(* Logix 5000 AddOnInstructionDefinition export Banner_LE_Param_v4; software revision 33.00; part 2 of 2 *)
(* tags used below, declared in another part *)
   LE : Banner_LE_v4;
   Port_Data : Banner_IOL_Port_v4;
   Port : DINT;
   Local_Control : DINT;
   Command_Being_Processed : BOOL;
   Update_Archive : BOOL;
   Index_Write_Control : DINT;
   Index_Write_Inprocess : INT;
   Inprocess_Index : DINT;
(* Banner_LE_Param_v4, continued *)

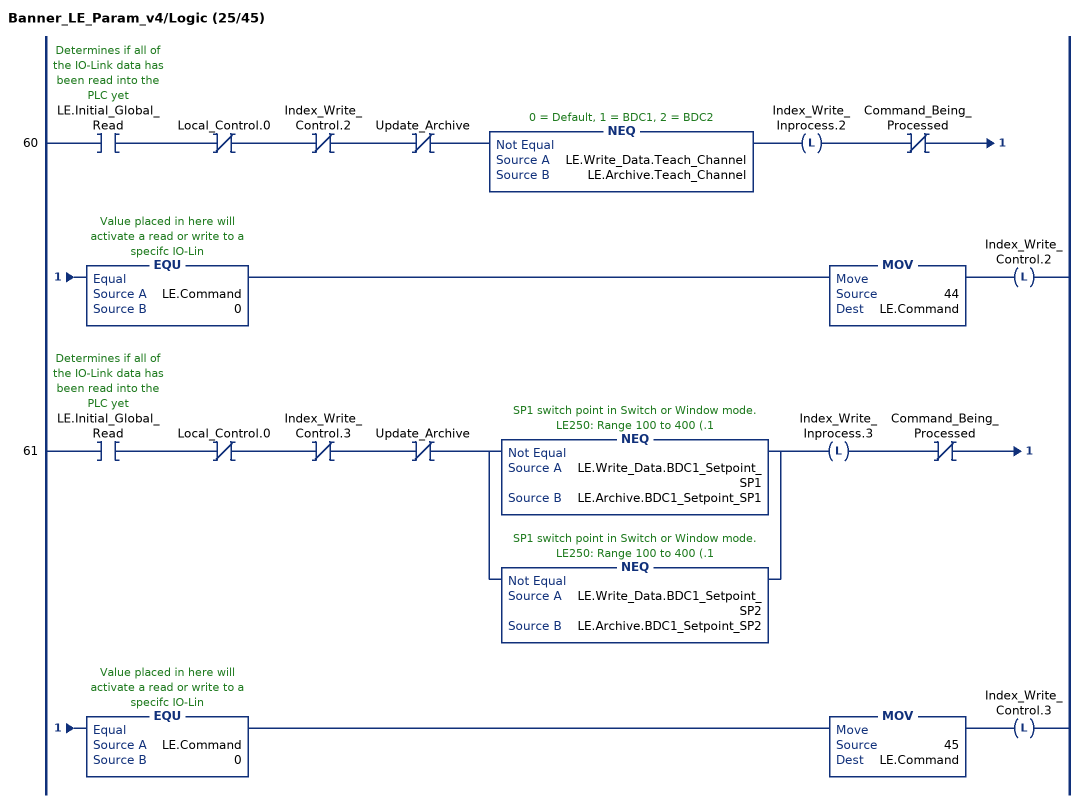
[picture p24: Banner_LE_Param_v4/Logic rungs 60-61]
   60: XIC(LE.Initial_Global_Read)XIO(Local_Control.0)XIO(Index_Write_Control.2)XIO(Update_Archive)NEQ(LE.Write_Data.Teach_Channel,LE.Archive.Teach_Channel)OTL(Index_Write_Inprocess.2)XIO(Command_Being_Processed)EQU(LE.Command,0)MOV(44,LE.Command)OTL(Index_Write_Control.2);
   61: XIC(LE.Initial_Global_Read)XIO(Local_Control.0)XIO(Index_Write_Control.3)XIO(Update_Archive)[NEQ(LE.Write_Data.BDC1_Setpoint_SP1,LE.Archive.BDC1_Setpoint_SP1) ,NEQ(LE.Write_Data.BDC1_Setpoint_SP2,LE.Archive.BDC1_Setpoint_SP2) ]OTL(Index_Write_Inprocess.3)XIO(Command_Being_Processed)EQU(LE.Command,0)MOV(45,LE.Command)OTL(Index_Write_Control.3);
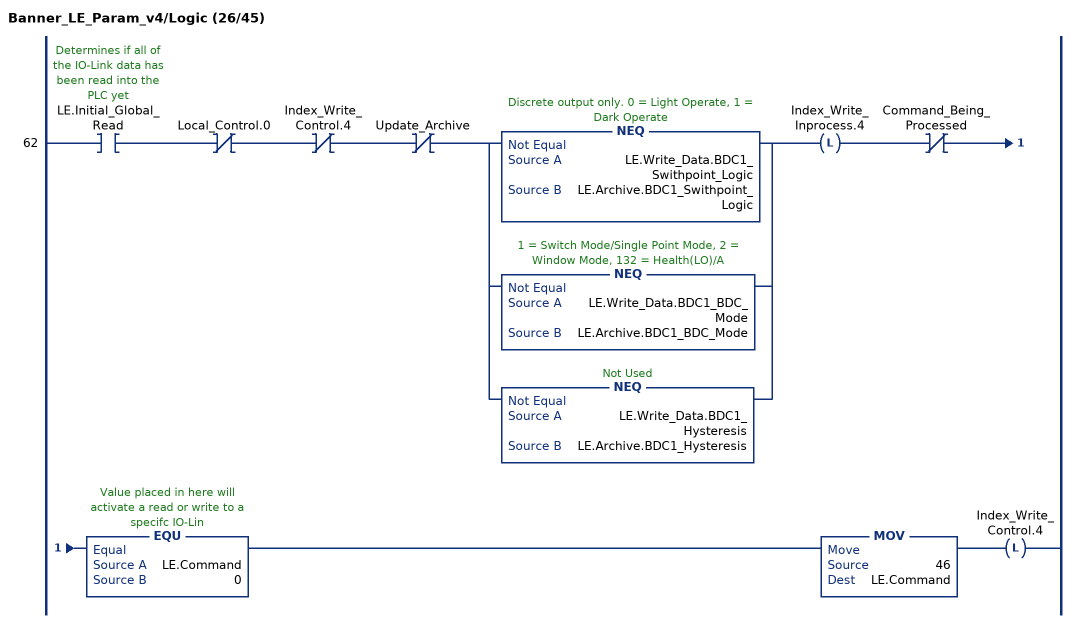
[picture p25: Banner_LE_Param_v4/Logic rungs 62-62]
   62: XIC(LE.Initial_Global_Read)XIO(Local_Control.0)XIO(Index_Write_Control.4)XIO(Update_Archive)[NEQ(LE.Write_Data.BDC1_Swithpoint_Logic,LE.Archive.BDC1_Swithpoint_Logic) ,NEQ(LE.Write_Data.BDC1_BDC_Mode,LE.Archive.BDC1_BDC_Mode) ,NEQ(LE.Write_Data.BDC1_Hysteresis,LE.Archive.BDC1_Hysteresis) ]OTL(Index_Write_Inprocess.4)XIO(Command_Being_Processed)EQU(LE.Command,0)MOV(46,LE.Command)OTL(Index_Write_Control.4);
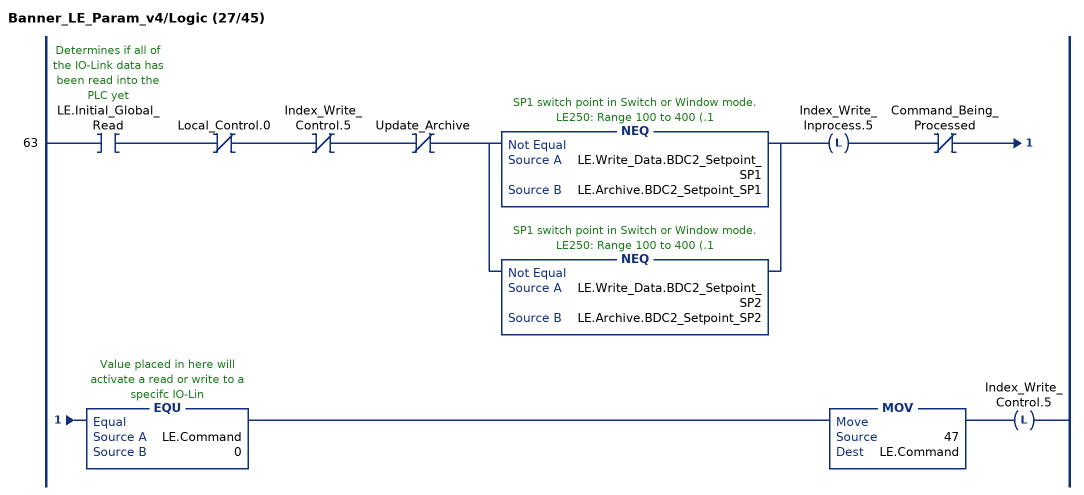
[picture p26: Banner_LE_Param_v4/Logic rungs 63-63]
   63: XIC(LE.Initial_Global_Read)XIO(Local_Control.0)XIO(Index_Write_Control.5)XIO(Update_Archive)[NEQ(LE.Write_Data.BDC2_Setpoint_SP1,LE.Archive.BDC2_Setpoint_SP1) ,NEQ(LE.Write_Data.BDC2_Setpoint_SP2,LE.Archive.BDC2_Setpoint_SP2) ]OTL(Index_Write_Inprocess.5)XIO(Command_Being_Processed)EQU(LE.Command,0)MOV(47,LE.Command)OTL(Index_Write_Control.5);
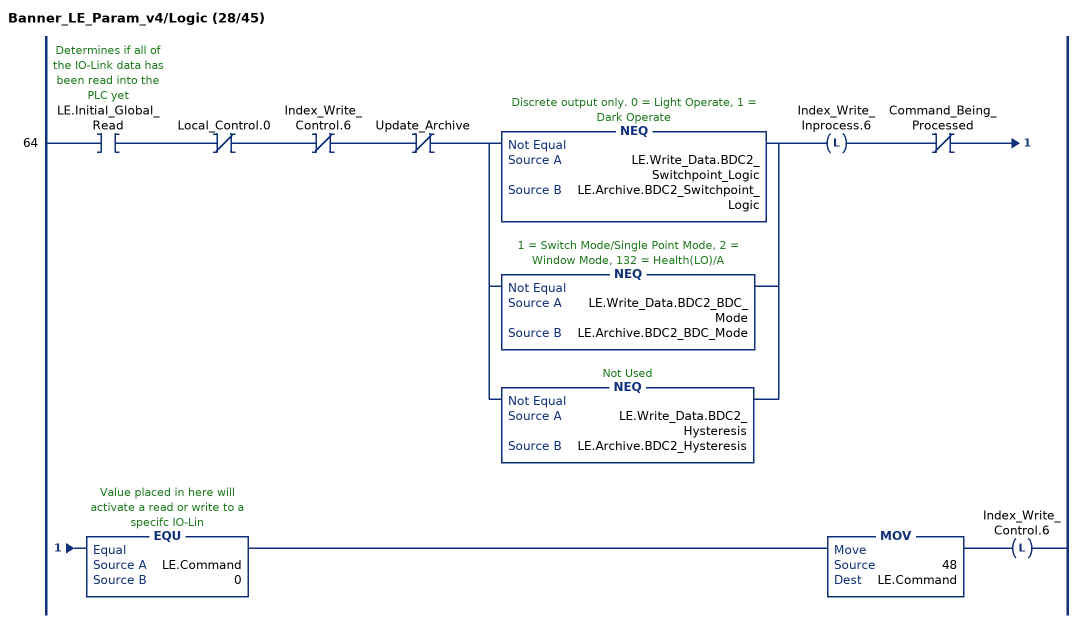
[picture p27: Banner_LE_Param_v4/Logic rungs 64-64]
   64: XIC(LE.Initial_Global_Read)XIO(Local_Control.0)XIO(Index_Write_Control.6)XIO(Update_Archive)[NEQ(LE.Write_Data.BDC2_Switchpoint_Logic,LE.Archive.BDC2_Switchpoint_Logic) ,NEQ(LE.Write_Data.BDC2_BDC_Mode,LE.Archive.BDC2_BDC_Mode) ,NEQ(LE.Write_Data.BDC2_Hysteresis,LE.Archive.BDC2_Hysteresis) ]OTL(Index_Write_Inprocess.6)XIO(Command_Being_Processed)EQU(LE.Command,0)MOV(48,LE.Command)OTL(Index_Write_Control.6);
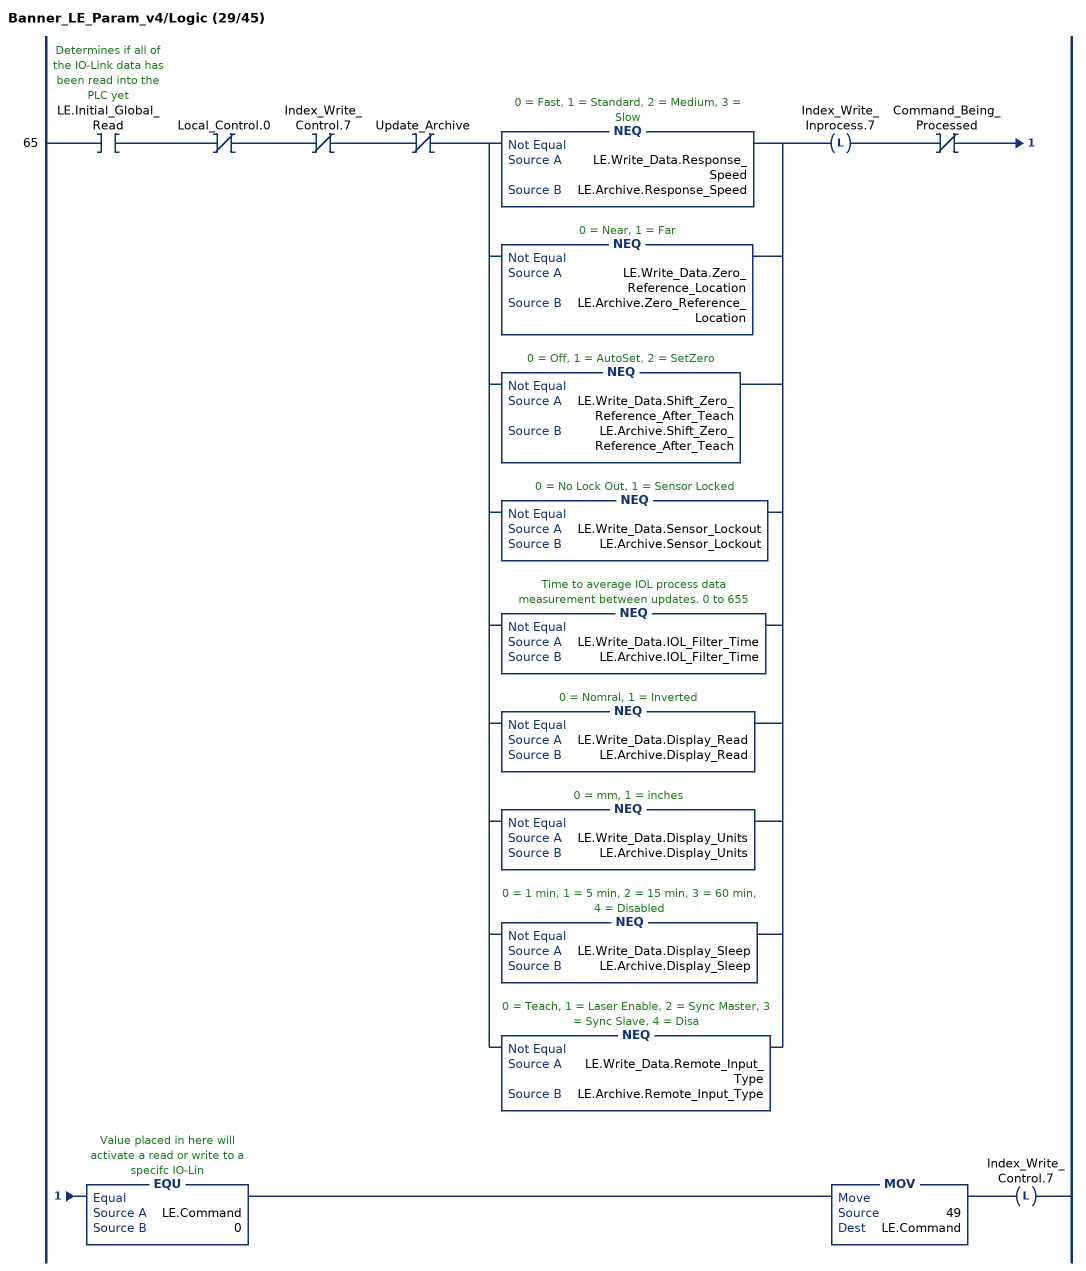
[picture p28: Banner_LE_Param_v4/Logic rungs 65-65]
   65: XIC(LE.Initial_Global_Read)XIO(Local_Control.0)XIO(Index_Write_Control.7)XIO(Update_Archive)[NEQ(LE.Write_Data.Response_Speed,LE.Archive.Response_Speed) ,NEQ(LE.Write_Data.Zero_Reference_Location,LE.Archive.Zero_Reference_Location) ,NEQ(LE.Write_Data.Shift_Zero_Reference_After_Teach,LE.Archive.Shift_Zero_Reference_After_Teach) ,NEQ(LE.Write_Data.Sensor_Lockout,LE.Archive.Sensor_Lockout) ,NEQ(LE.Write_Data.IOL_Filter_Time,LE.Archive.IOL_Filter_Time) ,NEQ(LE.Write_Data.Display_Read,LE.Archive.Display_Read) ,NEQ(LE.Write_Data.Display_Units,LE.Archive.Display_Units) ,NEQ(LE.Write_Data.Display_Sleep,LE.Archive.Display_Sleep) ,NEQ(LE.Write_Data.Remote_Input_Type,LE.Archive.Remote_Input_Type) ]OTL(Index_Write_Inprocess.7)XIO(Command_Being_Processed)EQU(LE.Command,0)MOV(49,LE.Command)OTL(Index_Write_Control.7);
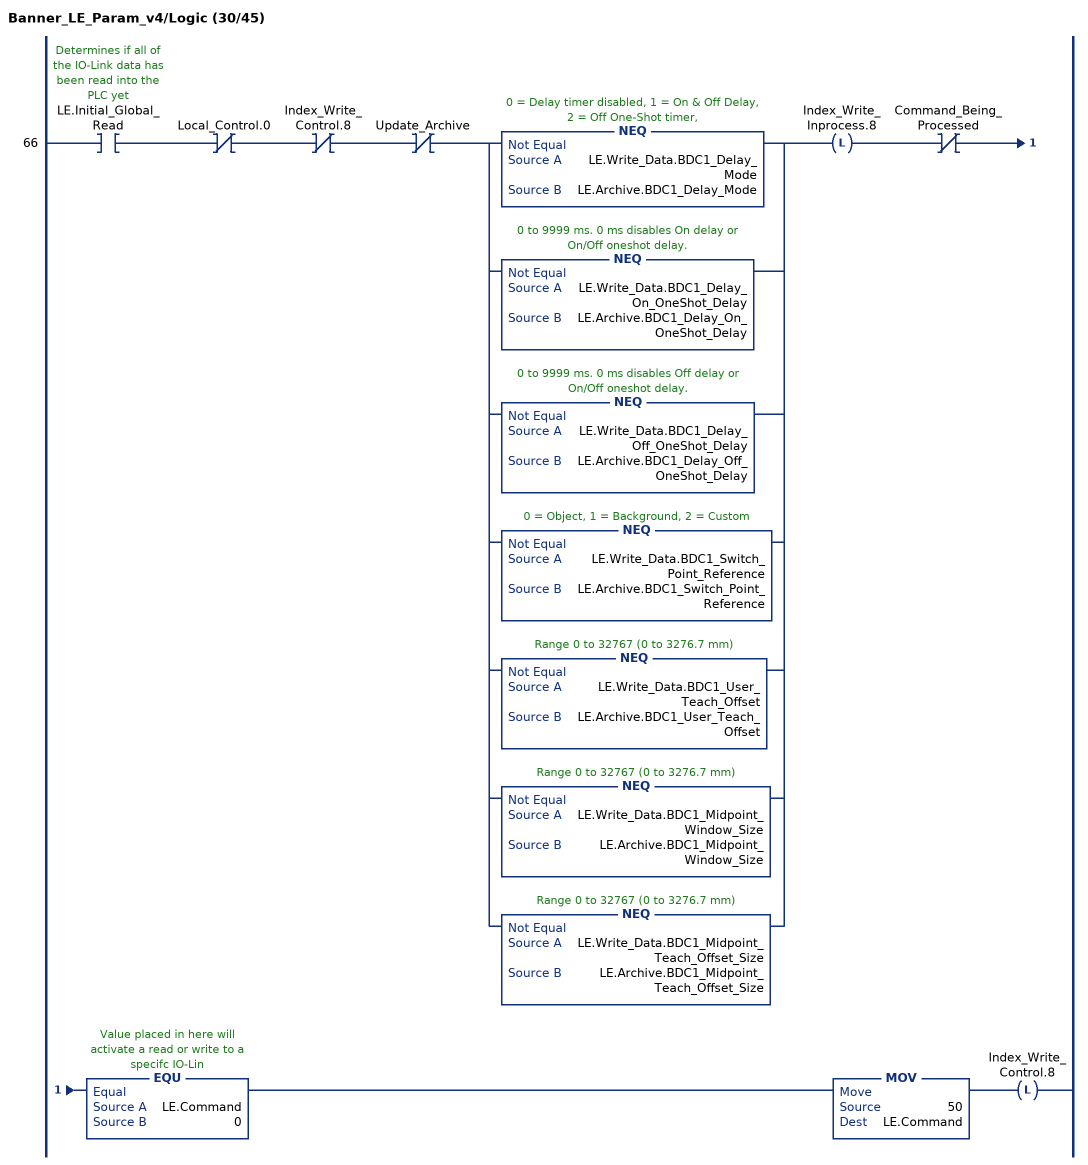
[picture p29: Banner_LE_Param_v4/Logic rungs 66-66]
   66: XIC(LE.Initial_Global_Read)XIO(Local_Control.0)XIO(Index_Write_Control.8)XIO(Update_Archive)[NEQ(LE.Write_Data.BDC1_Delay_Mode,LE.Archive.BDC1_Delay_Mode) ,NEQ(LE.Write_Data.BDC1_Delay_On_OneShot_Delay,LE.Archive.BDC1_Delay_On_OneShot_Delay) ,NEQ(LE.Write_Data.BDC1_Delay_Off_OneShot_Delay,LE.Archive.BDC1_Delay_Off_OneShot_Delay) ,NEQ(LE.Write_Data.BDC1_Switch_Point_Reference,LE.Archive.BDC1_Switch_Point_Reference) ,NEQ(LE.Write_Data.BDC1_User_Teach_Offset,LE.Archive.BDC1_User_Teach_Offset) ,NEQ(LE.Write_Data.BDC1_Midpoint_Window_Size,LE.Archive.BDC1_Midpoint_Window_Size) ,NEQ(LE.Write_Data.BDC1_Midpoint_Teach_Offset_Size,LE.Archive.BDC1_Midpoint_Teach_Offset_Size) ]OTL(Index_Write_Inprocess.8)XIO(Command_Being_Processed)EQU(LE.Command,0)MOV(50,LE.Command)OTL(Index_Write_Control.8);
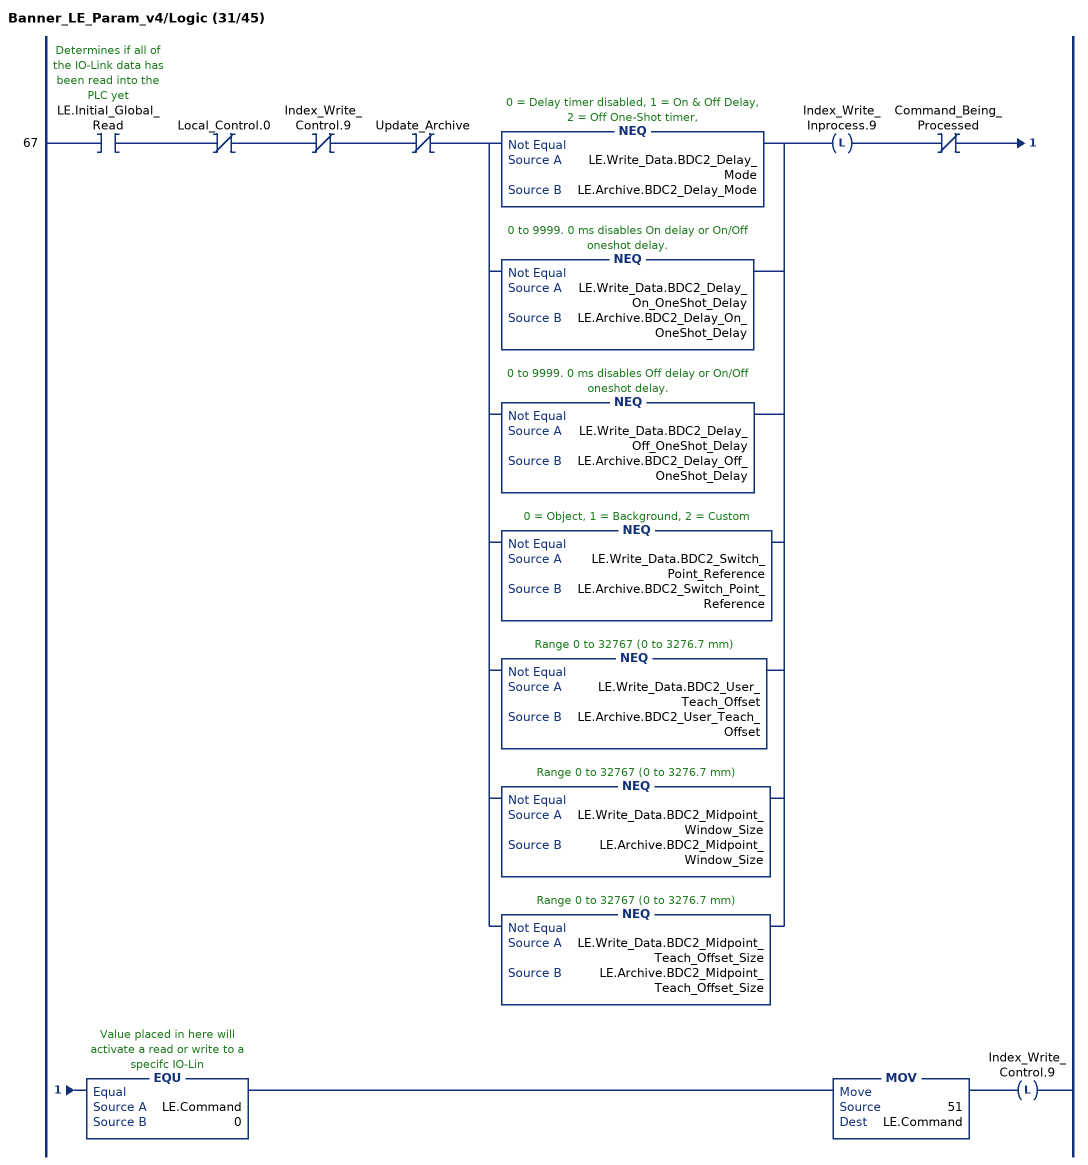
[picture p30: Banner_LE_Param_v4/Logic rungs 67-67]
   67: XIC(LE.Initial_Global_Read)XIO(Local_Control.0)XIO(Index_Write_Control.9)XIO(Update_Archive)[NEQ(LE.Write_Data.BDC2_Delay_Mode,LE.Archive.BDC2_Delay_Mode) ,NEQ(LE.Write_Data.BDC2_Delay_On_OneShot_Delay,LE.Archive.BDC2_Delay_On_OneShot_Delay) ,NEQ(LE.Write_Data.BDC2_Delay_Off_OneShot_Delay,LE.Archive.BDC2_Delay_Off_OneShot_Delay) ,NEQ(LE.Write_Data.BDC2_Switch_Point_Reference,LE.Archive.BDC2_Switch_Point_Reference) ,NEQ(LE.Write_Data.BDC2_User_Teach_Offset,LE.Archive.BDC2_User_Teach_Offset) ,NEQ(LE.Write_Data.BDC2_Midpoint_Window_Size,LE.Archive.BDC2_Midpoint_Window_Size) ,NEQ(LE.Write_Data.BDC2_Midpoint_Teach_Offset_Size,LE.Archive.BDC2_Midpoint_Teach_Offset_Size) ]OTL(Index_Write_Inprocess.9)XIO(Command_Being_Processed)EQU(LE.Command,0)MOV(51,LE.Command)OTL(Index_Write_Control.9);
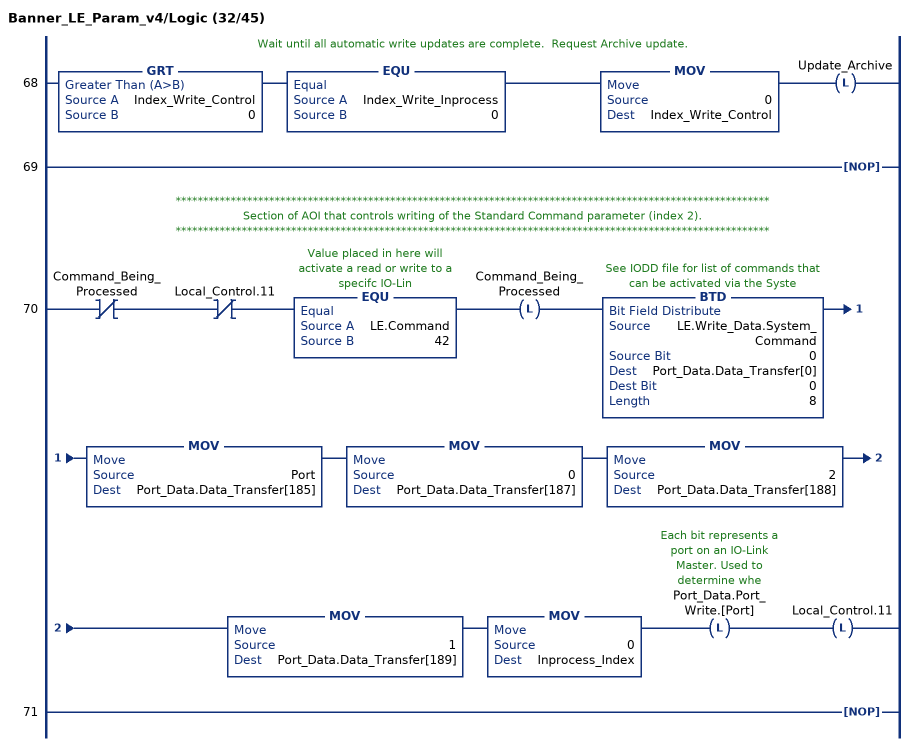
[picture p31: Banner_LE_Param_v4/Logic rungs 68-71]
   // Wait until all automatic write updates are complete.  Request Archive update.
   68: GRT(Index_Write_Control,0)EQU(Index_Write_Inprocess,0)MOV(0,Index_Write_Control)OTL(Update_Archive);
   69: NOP();
   // ************************************************************************************************************
   // Section of AOI that controls writing of the Standard Command parameter (index 2).
   // ************************************************************************************************************
   70: XIO(Command_Being_Processed)XIO(Local_Control.11)EQU(LE.Command,42)OTL(Command_Being_Processed)BTD(LE.Write_Data.System_Command,0,Port_Data.Data_Transfer[0],0,8)MOV(Port,Port_Data.Data_Transfer[185])MOV(0,Port_Data.Data_Transfer[187])MOV(2,Port_Data.Data_Transfer[188])MOV(1,Port_Data.Data_Transfer[189])MOV(0,Inprocess_Index)OTL(Port_Data.Port_Write.[Port])OTL(Local_Control.11);
   71: NOP();
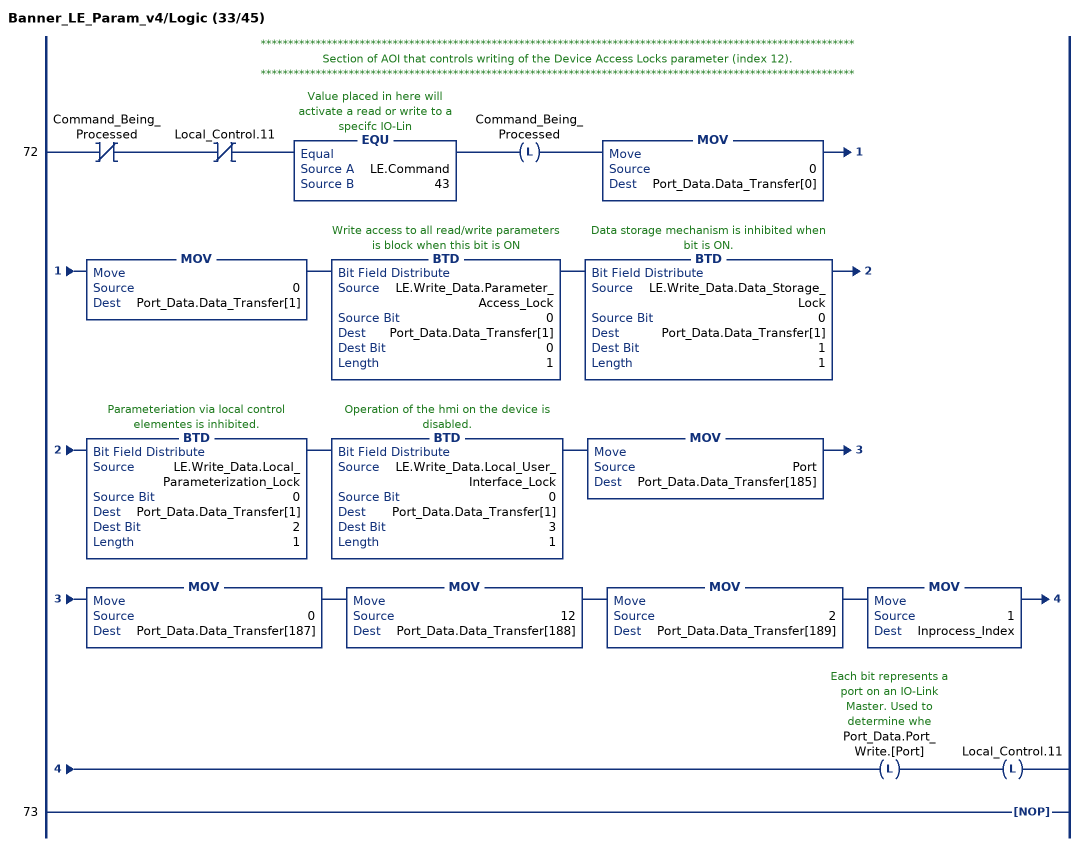
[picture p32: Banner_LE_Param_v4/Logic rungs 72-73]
   // ************************************************************************************************************
   // Section of AOI that controls writing of the Device Access Locks parameter (index 12).
   // ************************************************************************************************************
   72: XIO(Command_Being_Processed)XIO(Local_Control.11)EQU(LE.Command,43)OTL(Command_Being_Processed)MOV(0,Port_Data.Data_Transfer[0])MOV(0,Port_Data.Data_Transfer[1])BTD(LE.Write_Data.Parameter_Access_Lock,0,Port_Data.Data_Transfer[1],0,1)BTD(LE.Write_Data.Data_Storage_Lock,0,Port_Data.Data_Transfer[1],1,1)BTD(LE.Write_Data.Local_Parameterization_Lock,0,Port_Data.Data_Transfer[1],2,1)BTD(LE.Write_Data.Local_User_Interface_Lock,0,Port_Data.Data_Transfer[1],3,1)MOV(Port,Port_Data.Data_Transfer[185])MOV(0,Port_Data.Data_Transfer[187])MOV(12,Port_Data.Data_Transfer[188])MOV(2,Port_Data.Data_Transfer[189])MOV(1,Inprocess_Index)OTL(Port_Data.Port_Write.[Port])OTL(Local_Control.11);
   73: NOP();
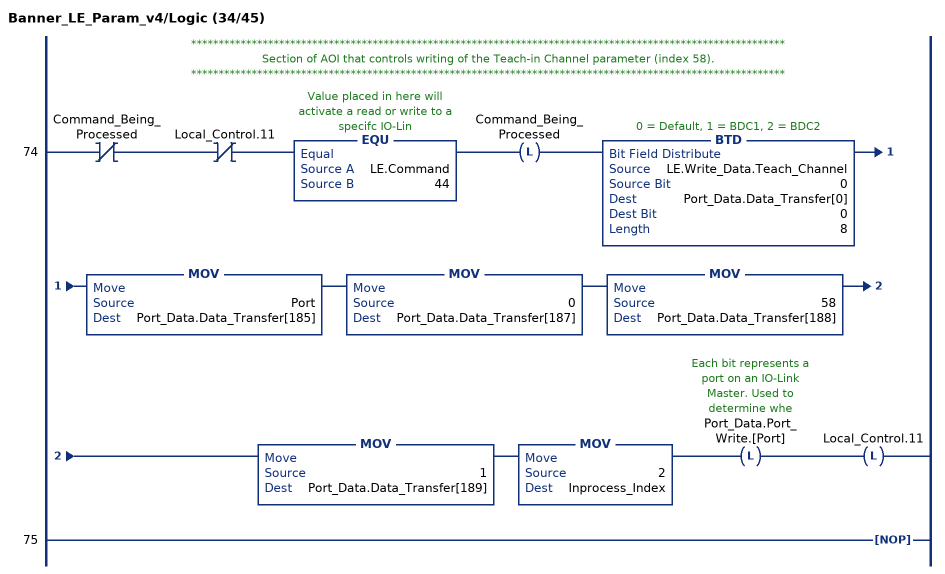
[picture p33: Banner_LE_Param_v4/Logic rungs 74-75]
   // ************************************************************************************************************
   // Section of AOI that controls writing of the Teach-in Channel parameter (index 58).
   // ************************************************************************************************************
   74: XIO(Command_Being_Processed)XIO(Local_Control.11)EQU(LE.Command,44)OTL(Command_Being_Processed)BTD(LE.Write_Data.Teach_Channel,0,Port_Data.Data_Transfer[0],0,8)MOV(Port,Port_Data.Data_Transfer[185])MOV(0,Port_Data.Data_Transfer[187])MOV(58,Port_Data.Data_Transfer[188])MOV(1,Port_Data.Data_Transfer[189])MOV(2,Inprocess_Index)OTL(Port_Data.Port_Write.[Port])OTL(Local_Control.11);
   75: NOP();
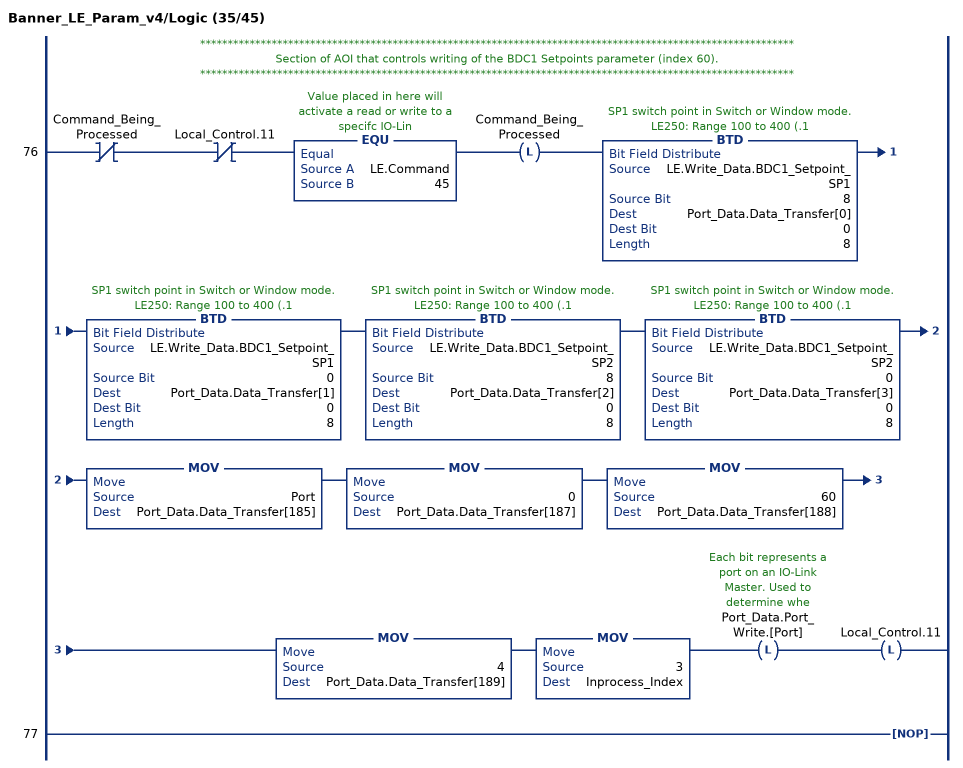
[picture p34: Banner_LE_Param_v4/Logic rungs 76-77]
   // ************************************************************************************************************
   // Section of AOI that controls writing of the BDC1 Setpoints parameter (index 60).
   // ************************************************************************************************************
   76: XIO(Command_Being_Processed)XIO(Local_Control.11)EQU(LE.Command,45)OTL(Command_Being_Processed)BTD(LE.Write_Data.BDC1_Setpoint_SP1,8,Port_Data.Data_Transfer[0],0,8)BTD(LE.Write_Data.BDC1_Setpoint_SP1,0,Port_Data.Data_Transfer[1],0,8)BTD(LE.Write_Data.BDC1_Setpoint_SP2,8,Port_Data.Data_Transfer[2],0,8)BTD(LE.Write_Data.BDC1_Setpoint_SP2,0,Port_Data.Data_Transfer[3],0,8)MOV(Port,Port_Data.Data_Transfer[185])MOV(0,Port_Data.Data_Transfer[187])MOV(60,Port_Data.Data_Transfer[188])MOV(4,Port_Data.Data_Transfer[189])MOV(3,Inprocess_Index)OTL(Port_Data.Port_Write.[Port])OTL(Local_Control.11);
   77: NOP();
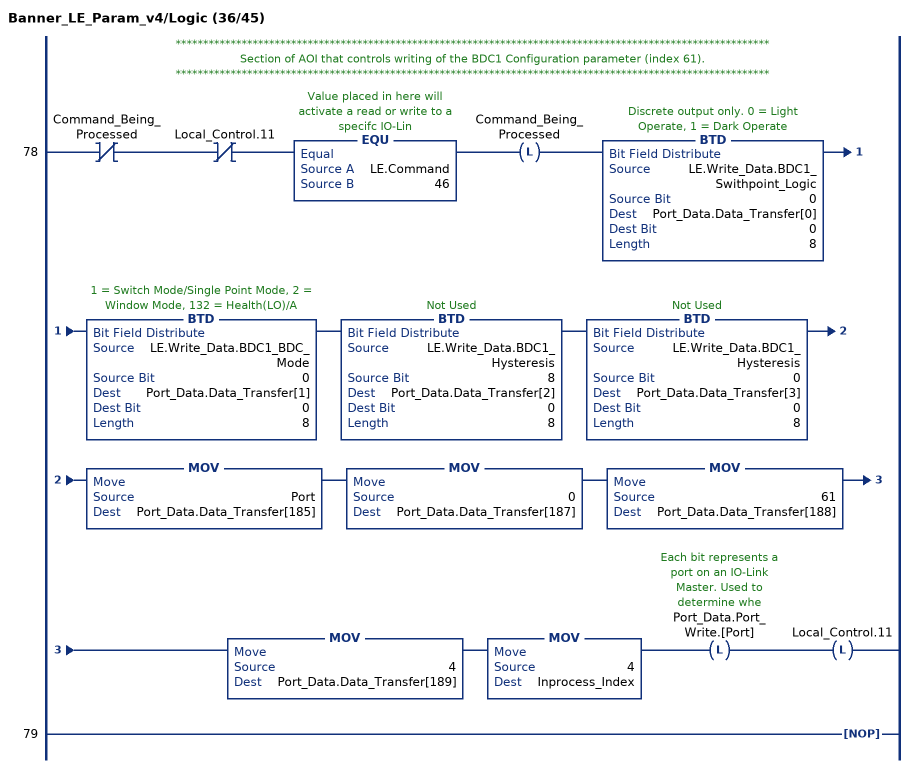
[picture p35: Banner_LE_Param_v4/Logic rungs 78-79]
   // ************************************************************************************************************
   // Section of AOI that controls writing of the BDC1 Configuration parameter (index 61).
   // ************************************************************************************************************
   78: XIO(Command_Being_Processed)XIO(Local_Control.11)EQU(LE.Command,46)OTL(Command_Being_Processed)BTD(LE.Write_Data.BDC1_Swithpoint_Logic,0,Port_Data.Data_Transfer[0],0,8)BTD(LE.Write_Data.BDC1_BDC_Mode,0,Port_Data.Data_Transfer[1],0,8)BTD(LE.Write_Data.BDC1_Hysteresis,8,Port_Data.Data_Transfer[2],0,8)BTD(LE.Write_Data.BDC1_Hysteresis,0,Port_Data.Data_Transfer[3],0,8)MOV(Port,Port_Data.Data_Transfer[185])MOV(0,Port_Data.Data_Transfer[187])MOV(61,Port_Data.Data_Transfer[188])MOV(4,Port_Data.Data_Transfer[189])MOV(4,Inprocess_Index)OTL(Port_Data.Port_Write.[Port])OTL(Local_Control.11);
   79: NOP();
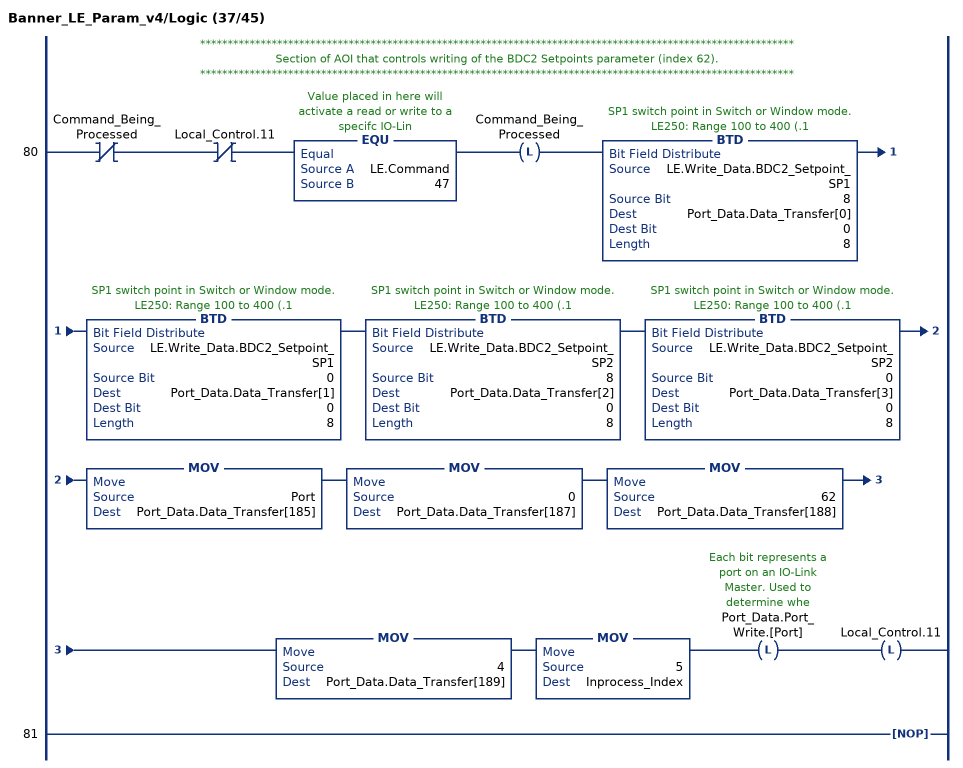
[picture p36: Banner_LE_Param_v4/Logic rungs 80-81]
   // ************************************************************************************************************
   // Section of AOI that controls writing of the BDC2 Setpoints parameter (index 62).
   // ************************************************************************************************************
   80: XIO(Command_Being_Processed)XIO(Local_Control.11)EQU(LE.Command,47)OTL(Command_Being_Processed)BTD(LE.Write_Data.BDC2_Setpoint_SP1,8,Port_Data.Data_Transfer[0],0,8)BTD(LE.Write_Data.BDC2_Setpoint_SP1,0,Port_Data.Data_Transfer[1],0,8)BTD(LE.Write_Data.BDC2_Setpoint_SP2,8,Port_Data.Data_Transfer[2],0,8)BTD(LE.Write_Data.BDC2_Setpoint_SP2,0,Port_Data.Data_Transfer[3],0,8)MOV(Port,Port_Data.Data_Transfer[185])MOV(0,Port_Data.Data_Transfer[187])MOV(62,Port_Data.Data_Transfer[188])MOV(4,Port_Data.Data_Transfer[189])MOV(5,Inprocess_Index)OTL(Port_Data.Port_Write.[Port])OTL(Local_Control.11);
   81: NOP();
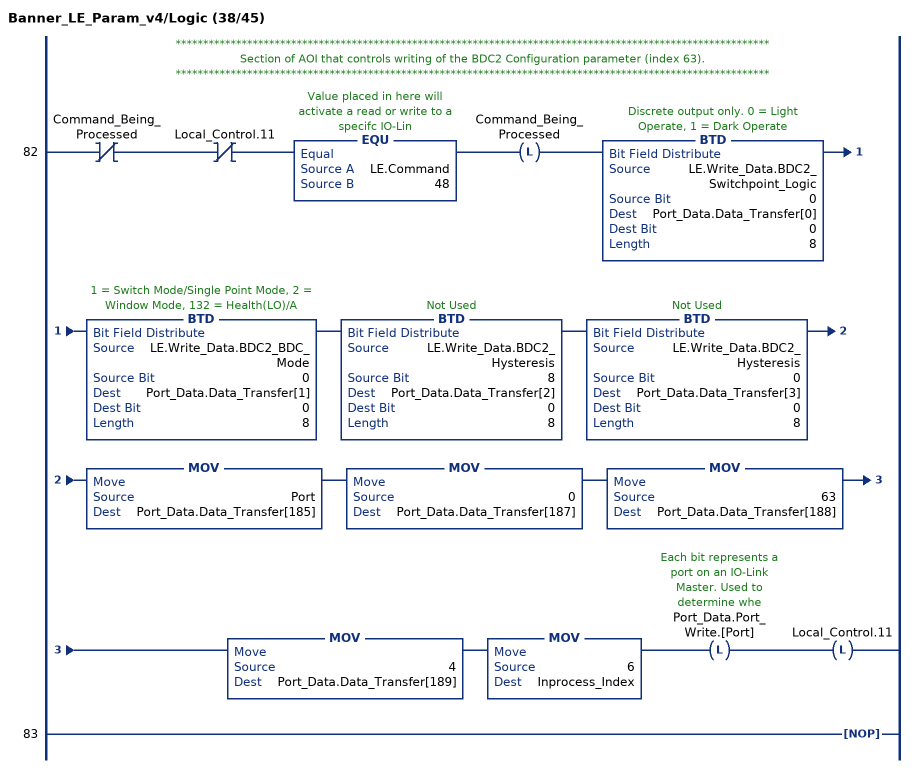
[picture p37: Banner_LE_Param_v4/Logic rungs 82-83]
   // ************************************************************************************************************
   // Section of AOI that controls writing of the BDC2 Configuration parameter (index 63).
   // ************************************************************************************************************
   82: XIO(Command_Being_Processed)XIO(Local_Control.11)EQU(LE.Command,48)OTL(Command_Being_Processed)BTD(LE.Write_Data.BDC2_Switchpoint_Logic,0,Port_Data.Data_Transfer[0],0,8)BTD(LE.Write_Data.BDC2_BDC_Mode,0,Port_Data.Data_Transfer[1],0,8)BTD(LE.Write_Data.BDC2_Hysteresis,8,Port_Data.Data_Transfer[2],0,8)BTD(LE.Write_Data.BDC2_Hysteresis,0,Port_Data.Data_Transfer[3],0,8)MOV(Port,Port_Data.Data_Transfer[185])MOV(0,Port_Data.Data_Transfer[187])MOV(63,Port_Data.Data_Transfer[188])MOV(4,Port_Data.Data_Transfer[189])MOV(6,Inprocess_Index)OTL(Port_Data.Port_Write.[Port])OTL(Local_Control.11);
   83: NOP();
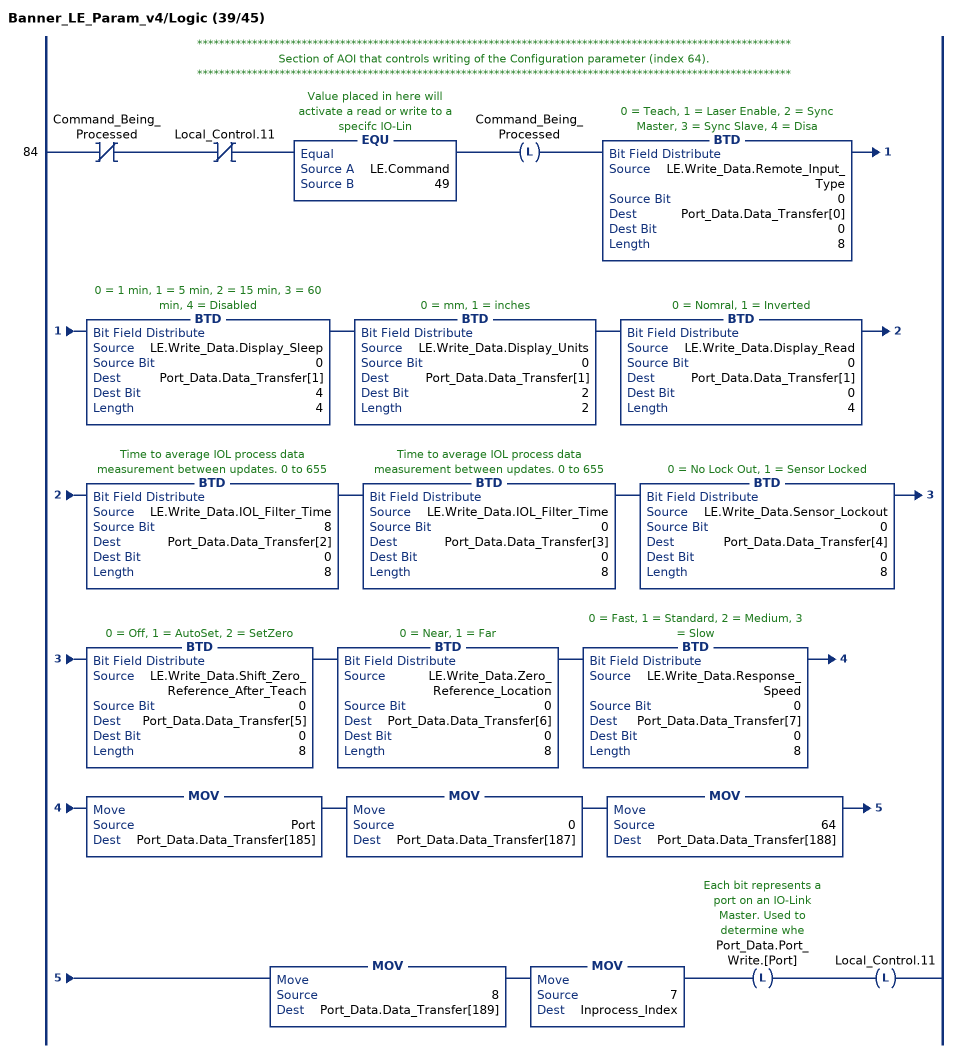
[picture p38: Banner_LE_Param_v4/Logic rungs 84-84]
   // ************************************************************************************************************
   // Section of AOI that controls writing of the Configuration parameter (index 64).
   // ************************************************************************************************************
   84: XIO(Command_Being_Processed)XIO(Local_Control.11)EQU(LE.Command,49)OTL(Command_Being_Processed)BTD(LE.Write_Data.Remote_Input_Type,0,Port_Data.Data_Transfer[0],0,8)BTD(LE.Write_Data.Display_Sleep,0,Port_Data.Data_Transfer[1],4,4)BTD(LE.Write_Data.Display_Units,0,Port_Data.Data_Transfer[1],2,2)BTD(LE.Write_Data.Display_Read,0,Port_Data.Data_Transfer[1],0,4)BTD(LE.Write_Data.IOL_Filter_Time,8,Port_Data.Data_Transfer[2],0,8)BTD(LE.Write_Data.IOL_Filter_Time,0,Port_Data.Data_Transfer[3],0,8)BTD(LE.Write_Data.Sensor_Lockout,0,Port_Data.Data_Transfer[4],0,8)BTD(LE.Write_Data.Shift_Zero_Reference_After_Teach,0,Port_Data.Data_Transfer[5],0,8)BTD(LE.Write_Data.Zero_Reference_Location,0,Port_Data.Data_Transfer[6],0,8)BTD(LE.Write_Data.Response_Speed,0,Port_Data.Data_Transfer[7],0,8)MOV(Port,Port_Data.Data_Transfer[185])MOV(0,Port_Data.Data_Transfer[187])MOV(64,Port_Data.Data_Transfer[188])MOV(8,Port_Data.Data_Transfer[189])MOV(7,Inprocess_Index)OTL(Port_Data.Port_Write.[Port])OTL(Local_Control.11);
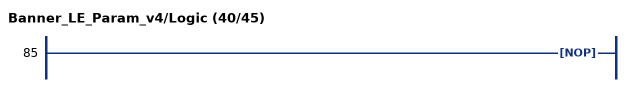
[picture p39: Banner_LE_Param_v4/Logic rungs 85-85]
   85: NOP();
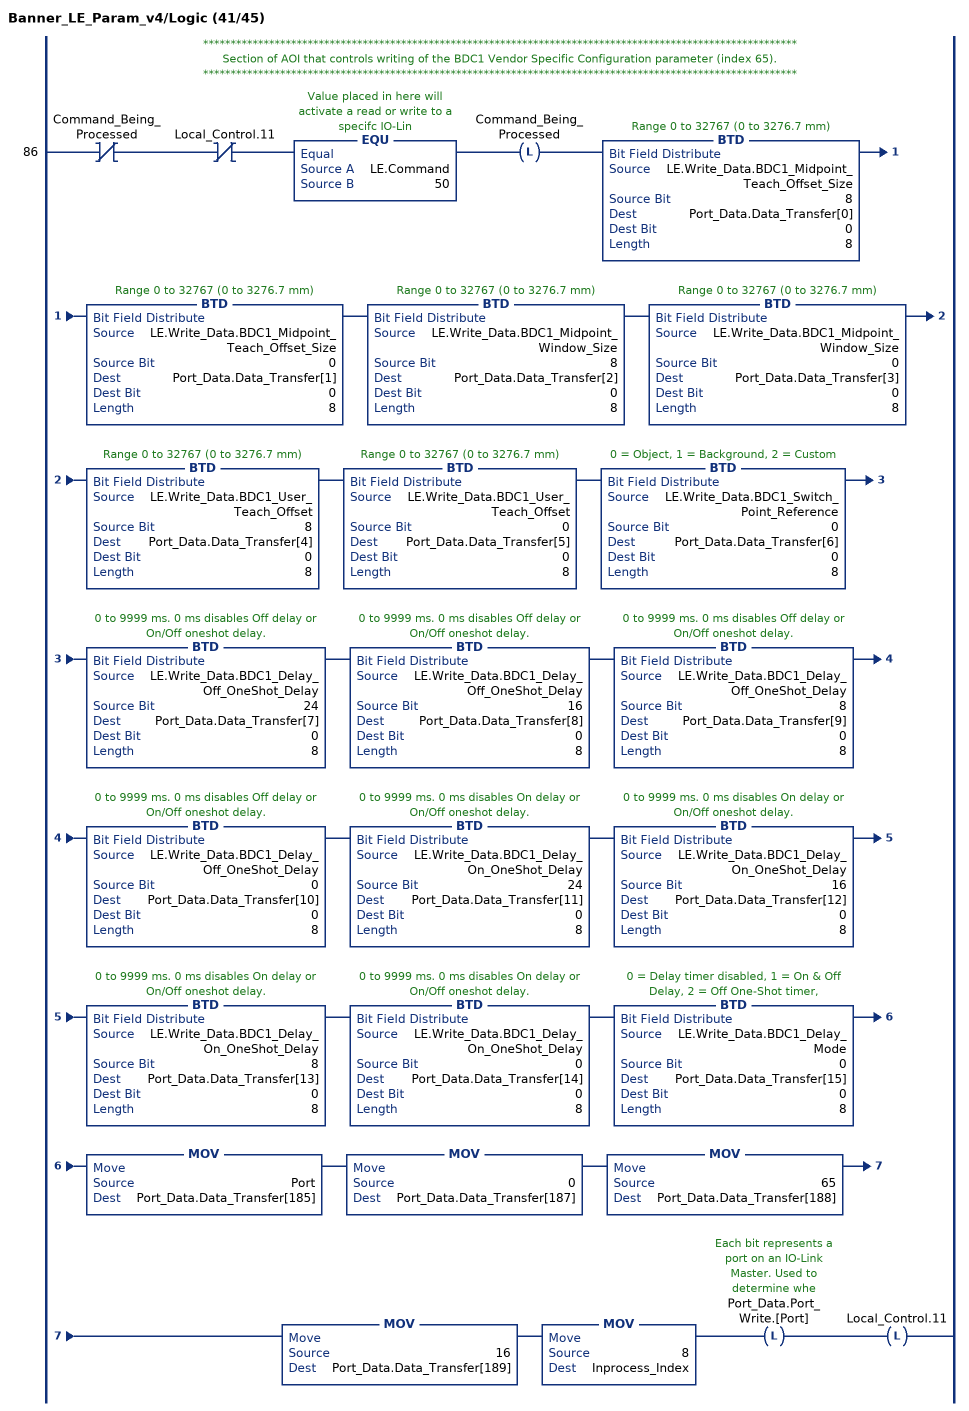
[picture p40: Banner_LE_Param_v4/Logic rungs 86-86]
   // ************************************************************************************************************
   // Section of AOI that controls writing of the BDC1 Vendor Specific Configuration parameter (index 65).
   // ************************************************************************************************************
   86: XIO(Command_Being_Processed)XIO(Local_Control.11)EQU(LE.Command,50)OTL(Command_Being_Processed)BTD(LE.Write_Data.BDC1_Midpoint_Teach_Offset_Size,8,Port_Data.Data_Transfer[0],0,8)BTD(LE.Write_Data.BDC1_Midpoint_Teach_Offset_Size,0,Port_Data.Data_Transfer[1],0,8)BTD(LE.Write_Data.BDC1_Midpoint_Window_Size,8,Port_Data.Data_Transfer[2],0,8)BTD(LE.Write_Data.BDC1_Midpoint_Window_Size,0,Port_Data.Data_Transfer[3],0,8)BTD(LE.Write_Data.BDC1_User_Teach_Offset,8,Port_Data.Data_Transfer[4],0,8)BTD(LE.Write_Data.BDC1_User_Teach_Offset,0,Port_Data.Data_Transfer[5],0,8)BTD(LE.Write_Data.BDC1_Switch_Point_Reference,0,Port_Data.Data_Transfer[6],0,8)BTD(LE.Write_Data.BDC1_Delay_Off_OneShot_Delay,24,Port_Data.Data_Transfer[7],0,8)BTD(LE.Write_Data.BDC1_Delay_Off_OneShot_Delay,16,Port_Data.Data_Transfer[8],0,8)BTD(LE.Write_Data.BDC1_Delay_Off_OneShot_Delay,8,Port_Data.Data_Transfer[9],0,8)BTD(LE.Write_Data.BDC1_Delay_Off_OneShot_Delay,0,Port_Data.Data_Transfer[10],0,8)BTD(LE.Write_Data.BDC1_Delay_On_OneShot_Delay,24,Port_Data.Data_Transfer[11],0,8)BTD(LE.Write_Data.BDC1_Delay_On_OneShot_Delay,16,Port_Data.Data_Transfer[12],0,8)BTD(LE.Write_Data.BDC1_Delay_On_OneShot_Delay,8,Port_Data.Data_Transfer[13],0,8)BTD(LE.Write_Data.BDC1_Delay_On_OneShot_Delay,0,Port_Data.Data_Transfer[14],0,8)BTD(LE.Write_Data.BDC1_Delay_Mode,0,Port_Data.Data_Transfer[15],0,8)MOV(Port,Port_Data.Data_Transfer[185])MOV(0,Port_Data.Data_Transfer[187])MOV(65,Port_Data.Data_Transfer[188])MOV(16,Port_Data.Data_Transfer[189])MOV(8,Inprocess_Index)OTL(Port_Data.Port_Write.[Port])OTL(Local_Control.11);
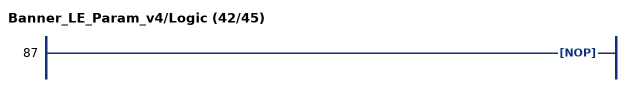
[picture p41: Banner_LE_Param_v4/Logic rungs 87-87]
   87: NOP();
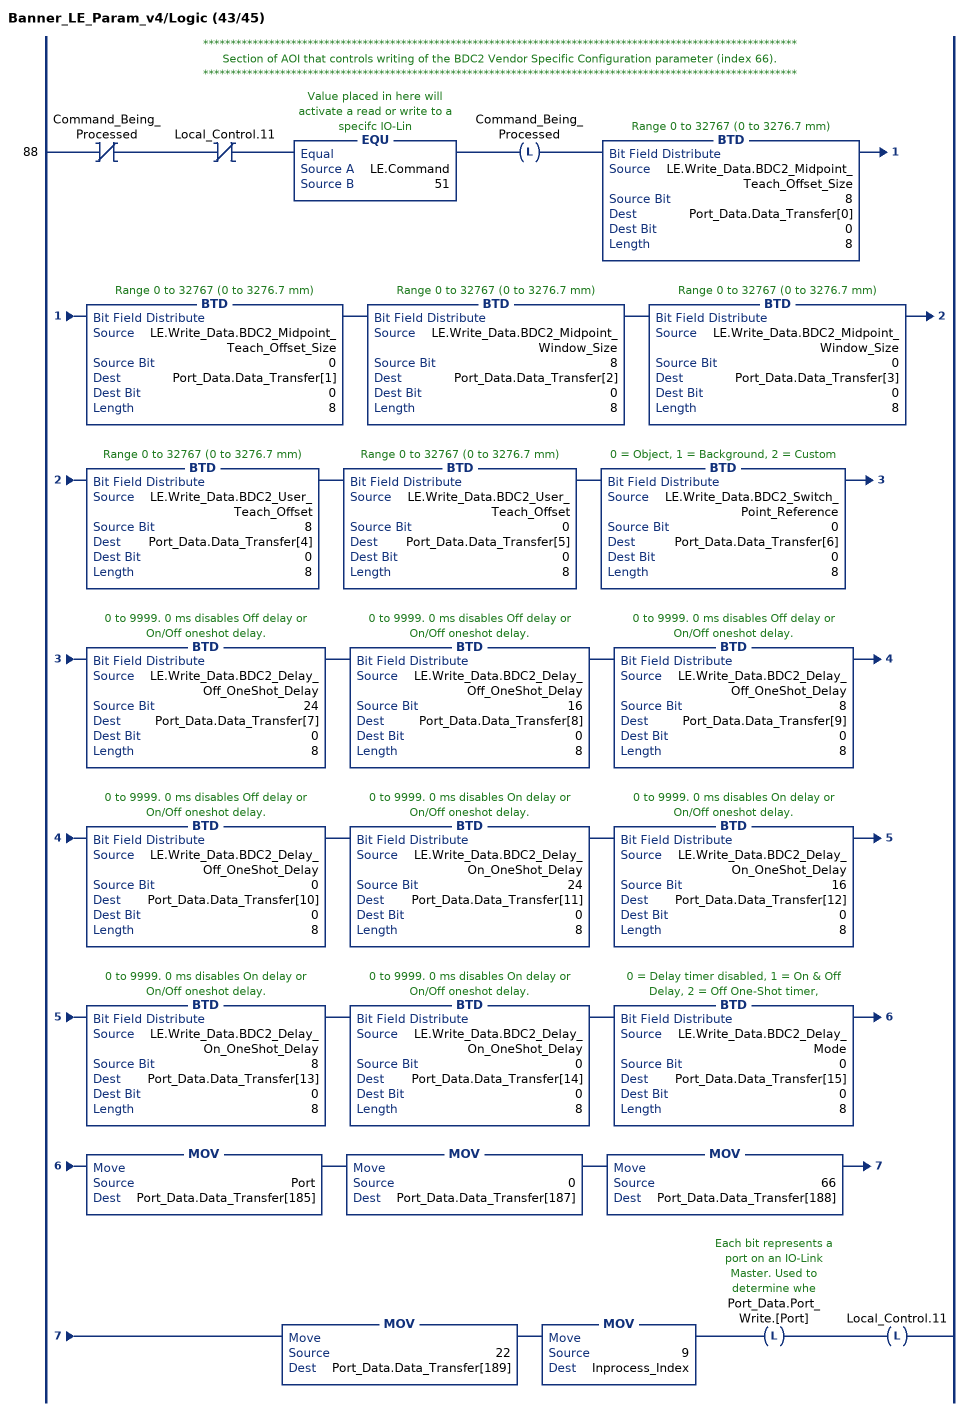
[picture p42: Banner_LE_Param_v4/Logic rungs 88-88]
   // ************************************************************************************************************
   // Section of AOI that controls writing of the BDC2 Vendor Specific Configuration parameter (index 66).
   // ************************************************************************************************************
   88: XIO(Command_Being_Processed)XIO(Local_Control.11)EQU(LE.Command,51)OTL(Command_Being_Processed)BTD(LE.Write_Data.BDC2_Midpoint_Teach_Offset_Size,8,Port_Data.Data_Transfer[0],0,8)BTD(LE.Write_Data.BDC2_Midpoint_Teach_Offset_Size,0,Port_Data.Data_Transfer[1],0,8)BTD(LE.Write_Data.BDC2_Midpoint_Window_Size,8,Port_Data.Data_Transfer[2],0,8)BTD(LE.Write_Data.BDC2_Midpoint_Window_Size,0,Port_Data.Data_Transfer[3],0,8)BTD(LE.Write_Data.BDC2_User_Teach_Offset,8,Port_Data.Data_Transfer[4],0,8)BTD(LE.Write_Data.BDC2_User_Teach_Offset,0,Port_Data.Data_Transfer[5],0,8)BTD(LE.Write_Data.BDC2_Switch_Point_Reference,0,Port_Data.Data_Transfer[6],0,8)BTD(LE.Write_Data.BDC2_Delay_Off_OneShot_Delay,24,Port_Data.Data_Transfer[7],0,8)BTD(LE.Write_Data.BDC2_Delay_Off_OneShot_Delay,16,Port_Data.Data_Transfer[8],0,8)BTD(LE.Write_Data.BDC2_Delay_Off_OneShot_Delay,8,Port_Data.Data_Transfer[9],0,8)BTD(LE.Write_Data.BDC2_Delay_Off_OneShot_Delay,0,Port_Data.Data_Transfer[10],0,8)BTD(LE.Write_Data.BDC2_Delay_On_OneShot_Delay,24,Port_Data.Data_Transfer[11],0,8)BTD(LE.Write_Data.BDC2_Delay_On_OneShot_Delay,16,Port_Data.Data_Transfer[12],0,8)BTD(LE.Write_Data.BDC2_Delay_On_OneShot_Delay,8,Port_Data.Data_Transfer[13],0,8)BTD(LE.Write_Data.BDC2_Delay_On_OneShot_Delay,0,Port_Data.Data_Transfer[14],0,8)BTD(LE.Write_Data.BDC2_Delay_Mode,0,Port_Data.Data_Transfer[15],0,8)MOV(Port,Port_Data.Data_Transfer[185])MOV(0,Port_Data.Data_Transfer[187])MOV(66,Port_Data.Data_Transfer[188])MOV(22,Port_Data.Data_Transfer[189])MOV(9,Inprocess_Index)OTL(Port_Data.Port_Write.[Port])OTL(Local_Control.11);
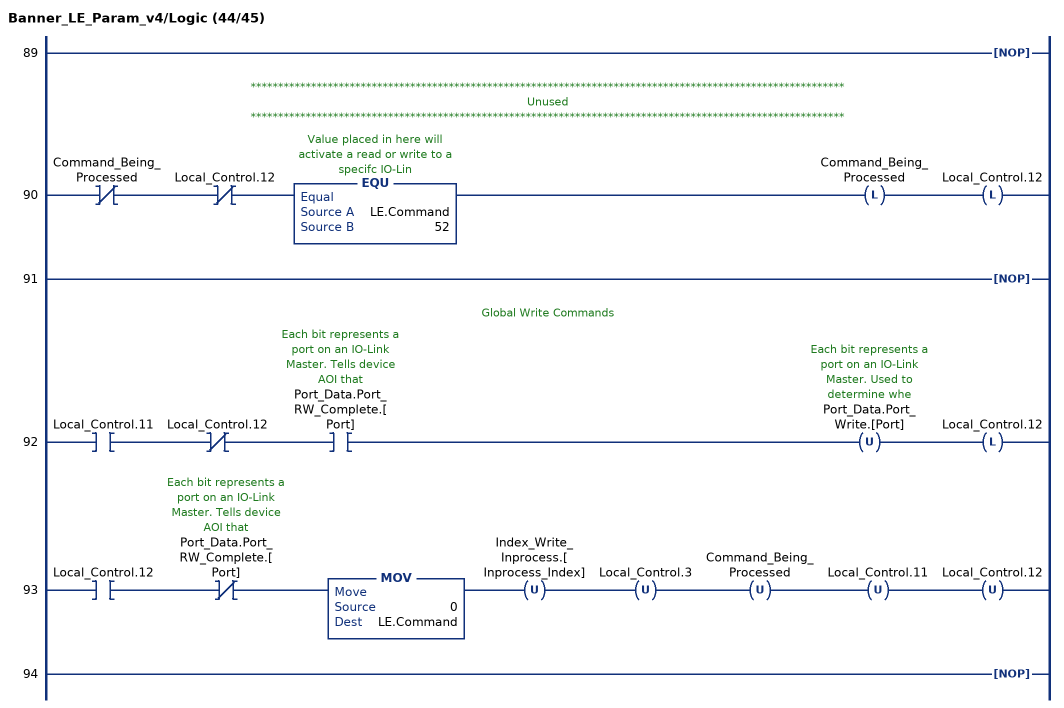
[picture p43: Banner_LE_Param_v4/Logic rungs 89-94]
   89: NOP();
   // ************************************************************************************************************
   // Unused
   // ************************************************************************************************************
   90: XIO(Command_Being_Processed)XIO(Local_Control.12)EQU(LE.Command,52)OTL(Command_Being_Processed)OTL(Local_Control.12);
   91: NOP();
   // Global Write Commands
   92: XIC(Local_Control.11)XIO(Local_Control.12)XIC(Port_Data.Port_RW_Complete.[Port])OTU(Port_Data.Port_Write.[Port])OTL(Local_Control.12);
   93: XIC(Local_Control.12)XIO(Port_Data.Port_RW_Complete.[Port])MOV(0,LE.Command)OTU(Index_Write_Inprocess.[Inprocess_Index])OTU(Local_Control.3)OTU(Command_Being_Processed)OTU(Local_Control.11)OTU(Local_Control.12);
   94: NOP();
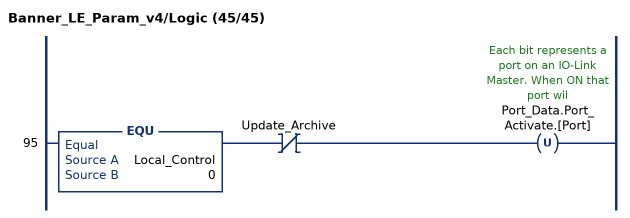
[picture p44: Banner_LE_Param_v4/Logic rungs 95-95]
   95: EQU(Local_Control,0)XIO(Update_Archive)OTU(Port_Data.Port_Activate.[Port]);
END_ROUTINE
END_ADD_ON_INSTRUCTION
